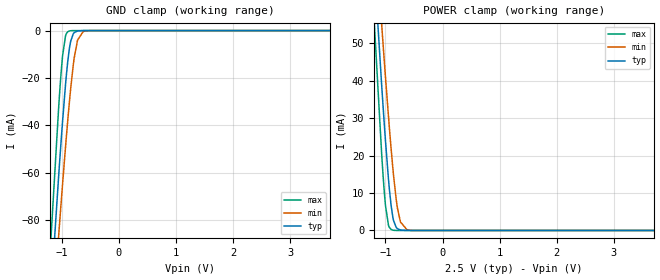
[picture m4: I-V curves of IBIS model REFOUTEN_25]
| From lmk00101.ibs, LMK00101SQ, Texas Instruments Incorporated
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|   Model REFOUTEN_25
[Model]   REFOUTEN_25
Model_type   Input
Vinl = 0.4
Vinh = 1.3
|   typ   min   max
C_comp   0.3093pF   0.3093pF   0.3093pF
[Voltage Range]   2.5   2.375   2.625
[Temperature Range]   45   125   -40
[Power Clamp Reference]   2.5   2.375   2.625
[GND Clamp Reference]   0   0   0
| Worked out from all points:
|   GND clamp passes 1 mA (typ) near -0.79 V on its own axis
|   POWER clamp passes 1 mA (typ) near -0.82 V on its own axis
[GND Clamp]
|   Voltage   I(typ)   I(min)   I(max)
-2.5V     -637.2mA   -600.8mA   -692.1mA
-1.21V    -119.2mA   -139mA     -96.66mA
-1.052V   -61.21mA   -86.45mA   -32.23mA
-1.045V   -58.59mA   -84.03mA   -29.51mA
-985mV    -38.45mA   -64.98mA   -10.78mA
-932.5mV  -22.7mA    -49.05mA   -2.191mA
-865mV    -7.577mA   -30.19mA   -157.9uA
-842.5mV  -4.524mA   -24.52mA   -59.03uA
-790mV    -1.101mA   -13.16mA   -4.75uA
-722.5mV  -153.3uA   -4.061mA   -164.7nA
-595mV    -1.786uA   -229uA     0A
4.992V    0A         0A         0A
[POWER Clamp]
|   Voltage   I(typ)   I(min)   I(max)
-2.5V     419.5mA    394.9mA    456.6mA
-1.218V   75.75mA    88.56mA    61.46mA
-1.067V   39.09mA    55.28mA    20.75mA
-1.06V    37.36mA    53.67mA    18.96mA
-1V       24.07mA    41.05mA    6.745mA
-947.5mV  13.82mA    30.55mA    1.418mA
-902.5mV  6.898mA    22.15mA    297.6uA
-857.5mV  2.631mA    14.62mA    49.35uA
-790mV    483.1uA    5.974mA    1.929uA
-737.5mV  113.4uA    2.296mA    140.3nA
-610mV    1.353uA    160.7uA    0A
4.992V    0A         0A         0A
